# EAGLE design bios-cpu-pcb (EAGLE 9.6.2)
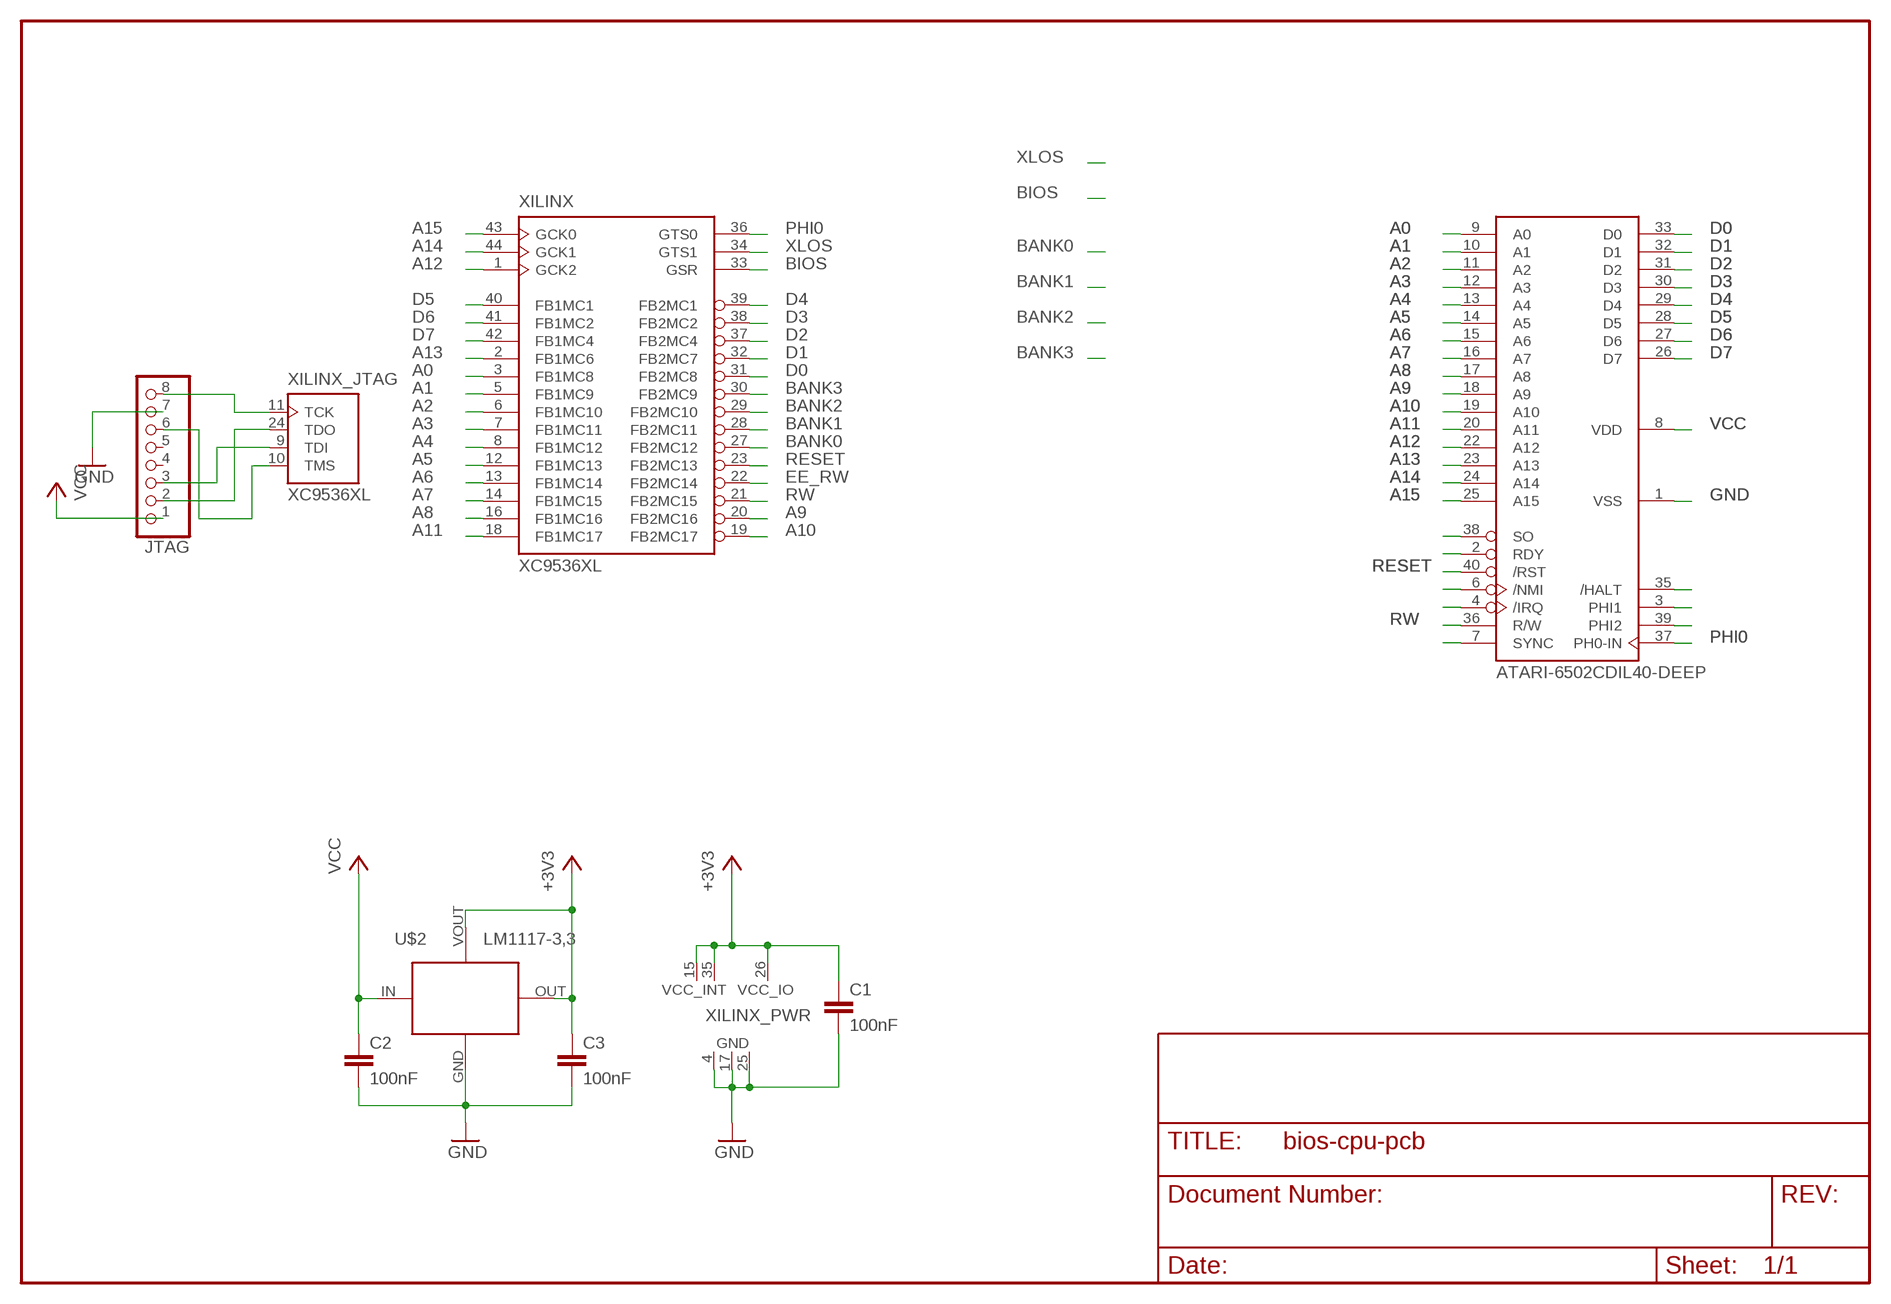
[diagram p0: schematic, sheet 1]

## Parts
C1  100nF  C-EUC0805  [C0805]
C2  100nF  C-EUC0805  [C0805]
C3  100nF  C-EUC0805  [C0805]
CPU1  ATARI-6502CDIL40-DEEP  [DIL40-DEEP]
JTAG  PINHD-1X8  [1X08]
U$2  LM1117-3,3  LM1117"  [SOT-223]
XILINX  XC9536XL  XC9536XL-VQ44  [VQ44]

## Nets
+3V3: C1.1 C3.1 U$2.OUT U$2.VOUT(CASE) XILINX.15(VCC_INT) XILINX.26(VCC_IO) XILINX.35(VCC_INT)
A0: CPU1.9(A0) XILINX.3(FB1MC8)
A1: CPU1.10(A1) XILINX.5(FB1MC9)
A2: CPU1.11(A2) XILINX.6(FB1MC10)
A3: CPU1.12(A3) XILINX.7(FB1MC11)
A4: CPU1.13(A4) XILINX.8(FB1MC12)
A5: CPU1.14(A5) XILINX.12(FB1MC13)
A6: CPU1.15(A6) XILINX.13(FB1MC14)
A7: CPU1.16(A7) XILINX.14(FB1MC15)
A8: CPU1.17(A8) XILINX.16(FB1MC16)
A9: CPU1.18(A9) XILINX.20(FB2MC16)
A10: CPU1.19(A10) XILINX.19(FB2MC17)
A11: CPU1.20(A11) XILINX.18(FB1MC17)
A12: CPU1.22(A12) XILINX.1(GCK2)
A13: CPU1.23(A13) XILINX.2(FB1MC6)
A14: CPU1.24(A14) XILINX.44(GCK1)
A15: CPU1.25(A15) XILINX.43(GCK0)
BANK0: XILINX.27(FB2MC12)
BANK1: XILINX.28(FB2MC11)
BANK2: XILINX.29(FB2MC10)
BANK3: XILINX.30(FB2MC9)
BIOS: XILINX.33(GSR)
D0: CPU1.33(D0) XILINX.31(FB2MC8)
D1: CPU1.32(D1) XILINX.32(FB2MC7)
D2: CPU1.31(D2) XILINX.37(FB2MC4)
D3: CPU1.30(D3) XILINX.38(FB2MC2)
D4: CPU1.29(D4) XILINX.39(FB2MC1)
D5: CPU1.28(D5) XILINX.40(FB1MC1)
D6: CPU1.27(D6) XILINX.41(FB1MC2)
D7: CPU1.26(D7) XILINX.42(FB1MC4)
EE_RW: XILINX.22(FB2MC14)
GND: C1.2 C2.2 C3.2 CPU1.1(VSS) JTAG.7 U$2.GND XILINX.4(GND) XILINX.17(GND) XILINX.25(GND)
N$1: JTAG.8 XILINX.11(TCK)
N$2: JTAG.2 XILINX.24(TDO)
N$3: JTAG.3 XILINX.9(TDI)
N$4: JTAG.6 XILINX.10(TMS)
N$5: CPU1.35(/HALT)
N$6: CPU1.3(PHI1)
N$7: CPU1.38(SO)
N$8: CPU1.2(RDY)
N$9: CPU1.6(/NMI)
N$10: CPU1.4(/IRQ)
N$11: CPU1.7(SYNC)
N$20: CPU1.39(PHI2)
PHI0: CPU1.37(PH0-IN) XILINX.36(GTS0)
RESET: CPU1.40(/RST) XILINX.23(FB2MC13)
RW: CPU1.36(R/W) XILINX.21(FB2MC15)
VCC: C2.1 CPU1.8(VDD) JTAG.1 U$2.IN
XLOS: XILINX.34(GTS1)
Unconnected: JTAG.4 JTAG.5

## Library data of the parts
C1-C3 = rcl:C-EU: CAPACITOR, European symbol
CPU1 = wf-atari:ATARI-6502C
JTAG = pinhead:PINHD-1X8: PIN HEADER
U$2 = lm1117:LM1117
XILINX = XC9500XLneu:XC9536XL-VQ44

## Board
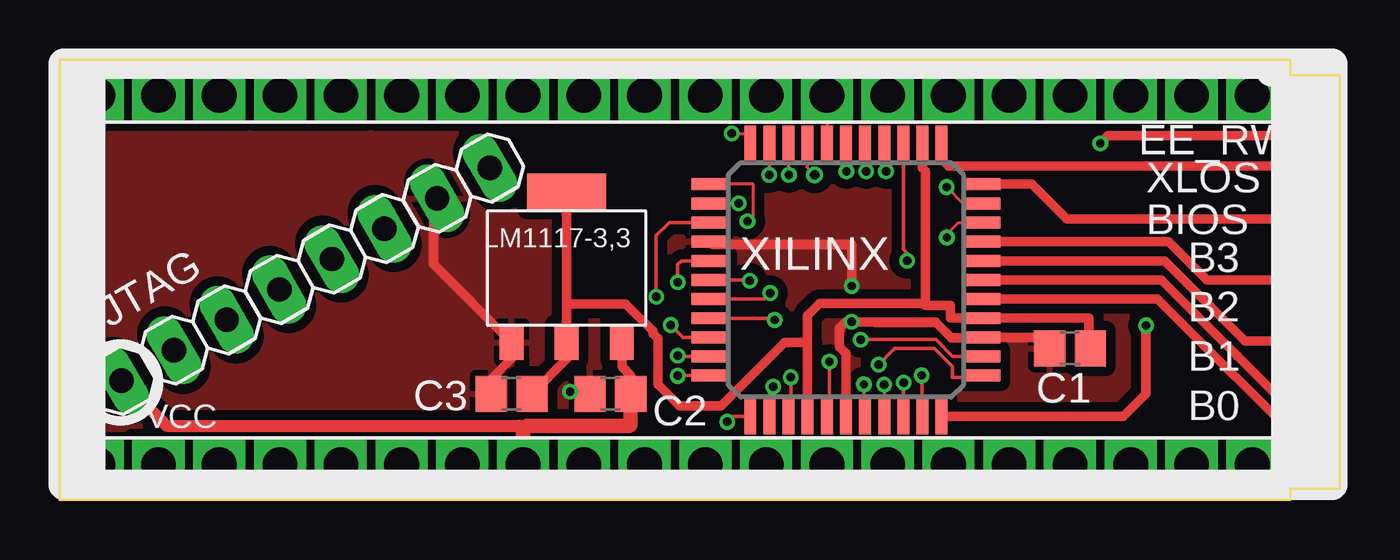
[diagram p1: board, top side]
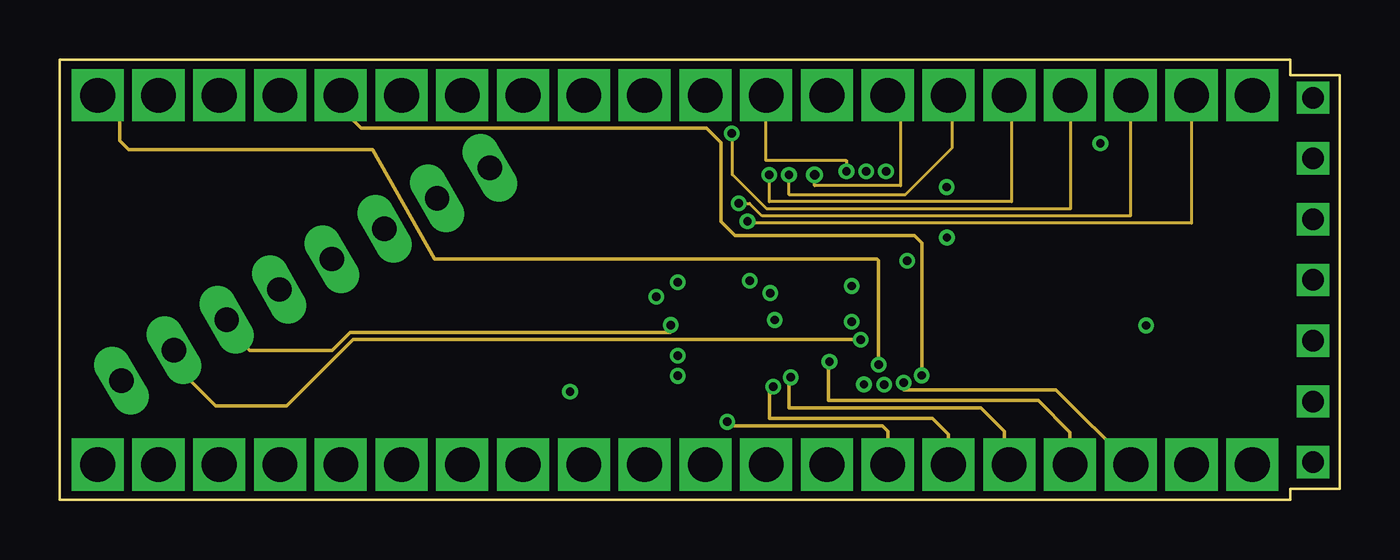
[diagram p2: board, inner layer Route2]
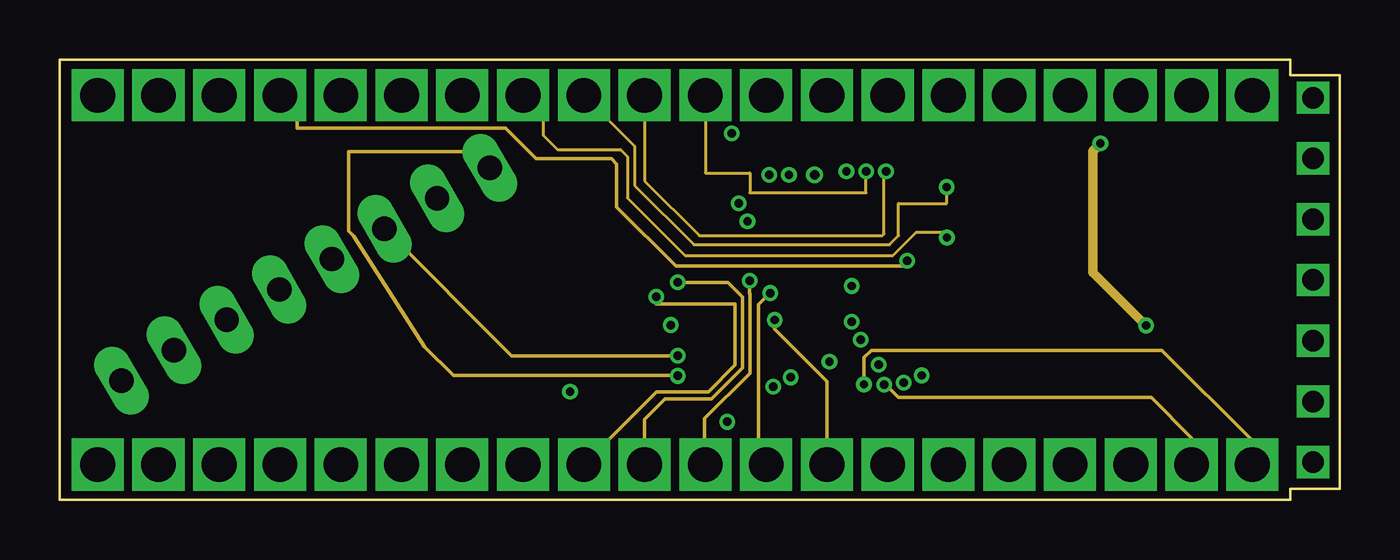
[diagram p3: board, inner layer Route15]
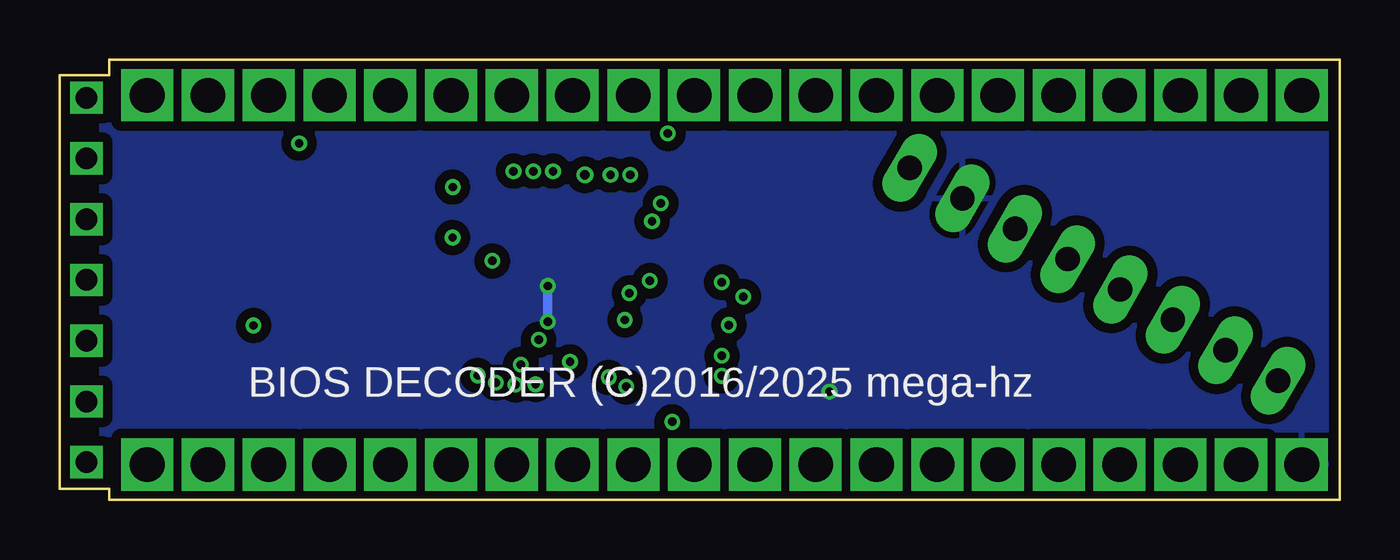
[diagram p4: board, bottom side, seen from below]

Size 53.49 x 18.41 mm. Coordinates in mm from the lower left corner, seen from the top.
Outline: 0,0 51.43,0 51.43,0.47 53.49,0.47 53.49,17.77 51.43,17.77 51.43,18.41 0,18.41 0,0
Copper layers (1+2*15+16): Top 0.035mm / dielectric 1.5mm / Route2 0.035mm / dielectric 0.15mm / Route15 0.035mm / dielectric 0.2mm / Bottom 0.035mm
Design rules "ITead_rule *": minimum track width 6mil, minimum drill 12mil, track to track 6mil, track to pad 6mil, pad to pad 6mil, via to via 6mil, smd to smd 0mil, copper to edge 10mil, drill to drill 10mil, minimum pad ring 10mil, minimum via ring 6mil, stop-mask expansion 2mil, vias tented up to drill 100mil, thermal gap 10mil

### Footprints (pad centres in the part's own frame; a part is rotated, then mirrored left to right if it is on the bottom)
C0805 = smd 1.3 x 1.5: 1 -0.85,0; 2 0.85,0
DIL40-DEEP = drill 1.45 pad 1.676 square: 1 -22.86,-7.72; 2 -20.32,-7.72; 3 -17.78,-7.72; 4 -15.24,-7.72; 5 -12.7,-7.72; 6 -10.16,-7.72; 7 -7.62,-7.72; 8 -5.08,-7.72; 9 -2.54,-7.72; 10 0,-7.72; 11 2.54,-7.72; 12 5.08,-7.72; 13 7.62,-7.72; 14 10.16,-7.72; 15 12.7,-7.72; 16 15.24,-7.72; 17 17.78,-7.72; 18 20.32,-7.72; 19 22.86,-7.72; 20 25.4,-7.72; 21 25.4,7.72; 22 22.86,7.72; 23 20.32,7.72; 24 17.78,7.72; 25 15.24,7.72; 26 12.7,7.72; 27 10.16,7.72; 28 7.62,7.72; 29 5.08,7.72; 30 2.54,7.72; 31 0,7.72; 32 -2.54,7.72; 33 -5.08,7.72; 34 -7.62,7.72; 35 -10.16,7.72; 36 -12.7,7.72; 37 -15.24,7.72; 38 -17.78,7.72; 39 -20.32,7.72; 40 -22.86,7.72
1X08 = drill 1.016 long: 1 -8.89,0; 2 -6.35,0; 3 -3.81,0; 4 -1.27,0; 5 1.27,0; 6 3.81,0; 7 6.35,0; 8 8.89,0
SOT-223 = smd 1 x 1.5: GND -2.3,-3; IN 2.3,-3; OUT 0,-3 | smd 3.3 x 1.5: VOUT 0,3.3
VQ44 = smd 1.5 x 0.5: 1 -5.7,4; 2 -5.7,3.2; 3 -5.7,2.4; 4 -5.7,1.6; 5 -5.7,0.8; 6 -5.7,0; 7 -5.7,-0.8; 8 -5.7,-1.6; 9 -5.7,-2.4; 10 -5.7,-3.2; 11 -5.7,-4; 23 5.7,-4; 24 5.7,-3.2; 25 5.7,-2.4; 26 5.7,-1.6; 27 5.7,-0.8; 28 5.7,0; 29 5.7,0.8; 30 5.7,1.6; 31 5.7,2.4; 32 5.7,3.2; 33 5.7,4 | smd 0.5 x 1.5: 12 -4,-5.7; 13 -3.2,-5.7; 14 -2.4,-5.7; 15 -1.6,-5.7; 16 -0.8,-5.7; 17 0,-5.7; 18 0.8,-5.7; 19 1.6,-5.7; 20 2.4,-5.7; 21 3.2,-5.7; 22 4,-5.7; 34 4,5.7; 35 3.2,5.7; 36 2.4,5.7; 37 1.6,5.7; 38 0.8,5.7; 39 0,5.7; 40 -0.8,5.7; 41 -1.6,5.7; 42 -2.4,5.7; 43 -3.2,5.7; 44 -4,5.7

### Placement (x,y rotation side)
C1  42.22,6.34 180 top
C2  23.01,4.44 180 top
C3  18.89,4.44 180 top
CPU1  24.44,9.2 0 top
JTAG  10.27,9.44 30 top
U$2  21.19,9.6 0 top
XILINX  32.86,9.2 0 top

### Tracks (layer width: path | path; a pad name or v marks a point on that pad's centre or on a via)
+3V3
  Top 0.406: C1.1 43.02,6.4 43.02,7.61 38.57,7.61 XILINX.26 37.23,7.6 37.23,8.13 36.18,8.13 36.18,8.21 | C3.1 21.19,5.89 U$2.OUT 21.19,8.2 | 21.19,8.2 U$2.VOUT | XILINX.15 31.26,6.58 | 31.26,6.58 31.26,7.71 31.76,8.21 36.18,8.21 | 36.18,8.21 36.18,13.75 36.06,13.87 XILINX.35 | 31.26,6.58 30.28,6.58 27.63,3.93 25.9,3.93 25,4.83 25,6.75 24.79,6.96 24.79,7.06 23.65,8.2 21.19,8.2
A0  (via drill 0.35)
  Top 0.152: v24.93,8.5 24.93,11.05 25.48,11.6 XILINX.3
  Route15 0.152: CPU1.9 24.95,4.53 27.1,4.53 28.23,5.65 28.23,8.2 24.93,8.2 v24.93,8.5
A1  (via drill 0.35)
  Top 0.152: v25.83,9.1 25.83,9.85 25.98,10 XILINX.5
  Route15 0.152: CPU1.10 24.44,3.36 25.3,4.22 27.23,4.22 28.53,5.53 28.53,8.5 27.93,9.1 v25.83,9.1
A2  (via drill 0.35)
  Top 0.152: XILINX.6 28.8,9.2 v28.83,9.17
  Route15 0.152: v28.83,9.17 28.83,8.63 28.84,8.62 28.84,5.29 26.95,3.4 26.95,1.51 CPU1.11
A3  (via drill 0.35)
  Top 0.152: v29.69,8.65 29.44,8.4 XILINX.7
  Route15 0.152: CPU1.12 29.2,1.8 29.2,8.17 v29.69,8.65
A4  (via drill 0.35)
  Top 0.152: XILINX.8 29.8,7.6 v29.88,7.53
  Route15 0.152: v29.88,7.53 29.88,7.15 32.06,4.97 CPU1.13
A5  (via drill 0.35)
  Top 0.152: v27.9,3.27 28.13,3.5 XILINX.12
  Route2 0.152: CPU1.14 34.6,2.88 34.38,3.1 28.15,3.1 27.99,3.27 v27.9,3.27
A6  (via drill 0.35)
  Top 0.152: v29.82,4.74 29.66,4.58 XILINX.13
  Route2 0.152: CPU1.15 37.14,2.74 36.47,3.41 29.65,3.41 29.65,4.58 v29.82,4.74
A7  (via drill 0.35)
  Top 0.152: v30.55,5.13 30.55,3.6 XILINX.14
  Route2 0.152: CPU1.16 39.48,1.69 39.48,2.88 38.5,3.85 30.48,3.85 30.48,5.05 v30.55,5.13
A8  (via drill 0.35)
  Top 0.152: v32.17,5.78 32.17,3.61 XILINX.16
  Route2 0.152: CPU1.17 42.22,2.83 40.9,4.16 32.13,4.16 32.13,5.74 v32.17,5.78
A9  (via drill 0.35)
  Top 0.152: v35.27,4.91 35.27,3.51 XILINX.20
  Route2 0.152: CPU1.18 41.64,4.6 36.26,4.6 36.25,4.6 35.81,4.6 35.8,4.6 35.28,4.6 35.27,4.62 v35.27,4.91
A10  (via drill 0.35)
  Top 0.152: v34.45,4.82 v34.46,4.81 XILINX.19
  Route15 0.152: CPU1.19 47.3,2.61 45.61,4.3 35.04,4.3 34.51,4.83 v34.45,4.83 v34.45,4.82
A11  (via drill 0.35)
  Top 0.152: v33.61,4.83 33.61,3.55 XILINX.18
  Route15 0.152: CPU1.20 49.84,2.49 46.07,6.26 33.91,6.26 33.61,5.96 v33.61,4.83
A12  (via drill 0.35)
  Top 0.127: v28.74,11.65 28.98,11.89 28.98,13.2 XILINX.1
  Route2 0.127: CPU1.22 47.3,11.58 28.82,11.58 v28.74,11.65
A13  (via drill 0.35)
  Top 0.127: XILINX.2 v28.38,12.4
  Route2 0.127: v28.38,12.4 28.83,12.4 29.35,11.88 44.76,11.88 CPU1.23
A14  (via drill 0.35)
  Top 0.127: v28.08,15.32 28.86,15.32 XILINX.44
  Route2 0.127: CPU1.24 42.25,16.92 42.25,12.18 29.54,12.18 28.12,13.6 28.12,15.29 v28.08,15.32
A15  (via drill 0.35)
  Top 0.127: v29.65,13.6 v29.66,13.6 XILINX.43
  Route2 0.127: CPU1.25 39.78,16.92 39.78,12.48 29.65,12.48 v29.65,13.6
BANK0  (via drill 0.9)
  Top 0.406: XILINX.27 45.88,8.4 52.38,1.9 v52.38,1.58
BANK1  (via drill 0.9)
  Top 0.406: XILINX.28 46.03,9.2 49.21,6.03 51.11,4.12 v52.38,4.12
BANK2  (via drill 0.9)
  Top 0.406: XILINX.29 46.18,10 48.1,8.09 49.53,6.66 v52.38,6.66
BANK3  (via drill 0.9)
  Top 0.406: XILINX.30 46.34,10.8 46.99,10.15 47.94,9.2 v52.38,9.2
BIOS  (via drill 0.9)
  Top 0.406: XILINX.33 40.64,13.2 42.1,11.74 v52.38,11.74
D0  (via drill 0.35)
  Top 0.127: v37.08,10.97 37.08,11.13 37.55,11.6 XILINX.31
  Route15 0.127: CPU1.33 20.2,16.08 20.2,15.25 20.8,14.65 23.43,14.65 23.73,14.35 23.73,12.63 26.13,10.23 34.83,10.23 35.8,11.2 37.01,11.2 37.08,11.13 v37.08,10.97
D1  (via drill 0.35)
  Top 0.127: v37.07,13.08 37.75,12.4 XILINX.32
  Route15 0.127: CPU1.32 24.03,14.8 24.03,13.15 26.5,10.68 34.68,10.68 35.05,11.05 35.05,12.4 37.07,12.4 v37.07,13.08
D2  (via drill 0.35)
  Top 0.127: XILINX.37 34.53,14.83 v34.53,13.75
  Route15 0.127: CPU1.31 24.44,13.34 26.73,11.05 34.38,11.05 34.45,11.13 34.45,13.6 34.42,13.64 v34.53,13.75
D3  (via drill 0.35)
  Top 0.127: v33.7,13.75 33.66,13.75 XILINX.38
  Route15 0.127: CPU1.30 26.98,13.68 28.84,13.68 28.84,12.85 33.7,12.85 v33.7,13.75
D4  (via drill 0.35)
  Top 0.127: v32.88,13.75 32.86,13.75 XILINX.39
  Route2 0.127: CPU1.29 29.5,16.92 29.5,14.2 32.88,14.2 v32.88,13.75
D5
  Top 0.127: CPU1.28 XILINX.40
D6  (via drill 0.4)
  Top 0.127: XILINX.41 31.23,14.87 31.23,13.92 v31.54,13.6
  Route2 0.127: CPU1.27 35.14,16.39 35.14,13.14 31.54,13.14 v31.54,13.6
D7  (via drill 0.35)
  Top 0.127: v30.48,13.6 30.46,13.6 XILINX.42
  Route2 0.127: CPU1.26 37.3,16.92 37.3,14.73 35.34,12.77 30.48,12.77 v30.48,13.6
EE_RW  (via drill 0.35, 0.9)
  Top 0.406: v52.38,16.82 52.38,16.47 51.15,15.23 43.81,15.23 v43.49,14.92 | XILINX.22 44.46,3.5 45.4,4.44 v45.4,7.3
  Route15 0.406: v45.4,7.3 43.17,9.52 43.17,14.6 v43.49,14.92
GND  (via drill 0.35)
  Top 0.152: C2.2 21.42,4.44 21.4,4.45 21.27,4.45 21.29,4.44 C2.2
  Top 0.406: C1.2 40.91,6.8 XILINX.25 38.53,6.78 37.26,6.78 36.59,7.45 v33.1,7.45 32.84,7.45 32.58,7.19 32.58,6.4 32.86,6.12 XILINX.17 | C3.2 18.04,5.06 18.89,5.91 U$2.GND 15.63,9.86 15.63,12.47 JTAG.7 | XILINX.4 27.28,10.68 33.1,10.68 v33.1,8.95
  Bottom 0.406: v33.1,8.95 v33.1,7.45
  other vias: 21.33,4.53
  pour Top (isolate 0.406): -0.32,18.73 51.75,18.73 51.75,-0.48 -0.32,-0.48
  pour Bottom (isolate 0.406): -0.32,18.73 51.75,18.73 51.75,-0.48 -0.32,-0.48
N$1  (via drill 0.35)
  Top 0.152: v25.83,5.19 25.84,5.2 XILINX.11
  Route15 0.152: JTAG.8 17.29,14.56 12.08,14.56 12.08,11.25 12.29,11.04 15.25,6.41 16.45,5.2 25.83,5.2 v25.83,5.19
N$2  (via drill 0.35)
  Top 0.152: XILINX.24 37.31,6 36.61,6.7 v33.48,6.7
  Route2 0.152: v33.48,6.7 12.25,6.7 9.48,3.93 6.51,3.93 4.77,5.67 JTAG.2
N$3  (via drill 0.35)
  Top 0.152: v25.53,7.32 26.05,6.8 XILINX.9
  Route2 0.152: JTAG.3 6.97,7.22 7.93,6.25 11.37,6.25 12.13,7.01 25.53,7.01 v25.53,7.32
N$4  (via drill 0.35)
  Top 0.152: v25.82,6.03 25.85,6 XILINX.10
  Route15 0.152: JTAG.6 18.88,6.03 v25.82,6.03
PHI0  (via drill 0.35)
  Top 0.152: v35.41,10 35.41,10.32 35.26,10.48 XILINX.36
  Route15 0.152: CPU1.37 9.93,16.2 9.93,15.55 18.63,15.55 19.9,14.28 23.05,14.28 23.28,14.05 23.28,12.25 25.75,9.78 35.28,9.78 35.5,10 v35.41,10
RESET  (via drill 0.35)
  Top 0.152: v34.22,5.66 34.89,6.33 36.55,6.33 37.3,5.58 37.3,5.13 38.48,5.13 XILINX.23
  Route2 0.152: CPU1.40 2.5,16 2.5,15.03 2.88,14.65 13.07,14.65 15.67,10.08 34.15,10.08 34.22,10.01 v34.22,5.66
RW  (via drill 0.35)
  Top 0.152: v36.03,5.21 36.03,3.53 XILINX.21
  Route2 0.152: CPU1.36 11.74,16.4 12.59,15.55 27.03,15.55 27.63,14.95 27.63,11.65 28.23,11.05 35.73,11.05 36.03,10.75 v36.03,5.21
VCC
  Top 0.406: C2.1 23.86,5.22 23.49,5.59 U$2.IN
  Top 0.508: JTAG.1 4.46,3.1 19.2,3.1 19.36,2.94
  Top 0.61: CPU1.8 19.36,2.94 19.53,3.1 23.8,3.1 23.86,3.16 C2.1
XLOS  (via drill 0.9)
  Top 0.406: XILINX.34 36.86,14.25 37.14,13.96 49.84,13.96 50,13.96 52.06,13.96 v52.38,14.28

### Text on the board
tPlace: EE_RW | XLOS | BIOS | B3 | B2 | B1 | B0 | VCC
bPlace: BIOS DECODER (C)2016/2025 mega-hz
